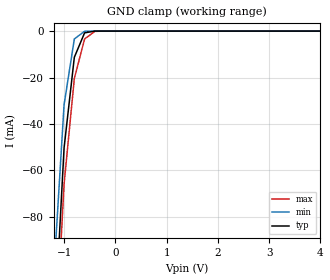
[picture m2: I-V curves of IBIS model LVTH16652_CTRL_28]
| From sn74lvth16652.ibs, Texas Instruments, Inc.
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|   Model LVTH16652 Input_CTRL_28
[Model]   LVTH16652_CTRL_28
Model_type  Input
Polarity   Inverting
Vinl = 0.8V
Vinh = 2.0V
| variable   typ   min   max
C_comp   4pf   NA   NA
[Temperature Range]   40   -25   100
| Ambient temperature   25   -40   85
[Voltage range]   2.8   2.7   2.9
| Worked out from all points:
|   GND clamp passes 1 mA (typ) near -0.60 V on its own axis
[GND Clamp]
|   Voltage   I(typ)   I(min)   I(max)
-5V       -2.458A    -2.828A    -2.149A
-1.2V     -133.5mA   -104.4mA   -149.5mA
-1V       -50.3mA    -31.7mA    -65.89mA
-800mV    -11.29mA   -3.392mA   -20.43mA
-600mV    -765.2uA   -68.88uA   -3.39mA
-400mV    -2.612uA   -87nA      -121.2uA
5V        -24.32pA   659.7nA    418pA
